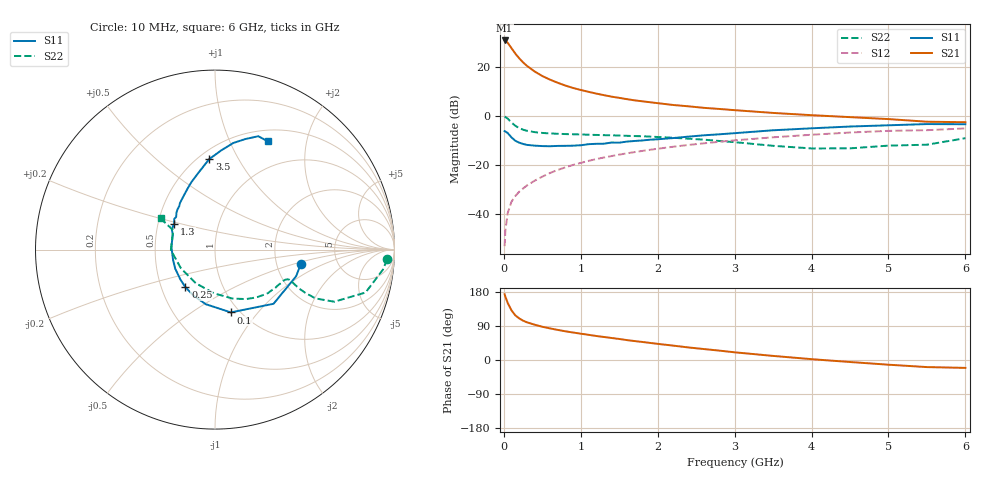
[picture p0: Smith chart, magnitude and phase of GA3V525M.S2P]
! Infineon Technologies  Discrete & RF Semiconductors
! BF775
! Si NPN RF Bipolar Junction Transistor in SOT23
! VCE = 3.5 V  IC = 25 mA
! Common Emitter S-Parameters:  May  1996
# GHz  S  MA  R  50
!  f  S11  S21  S12  S22
! GHz  MAG  ANG  MAG  ANG  MAG  ANG  MAG  ANG
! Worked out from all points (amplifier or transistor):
!   36 points, 10 MHz to 6 GHz, reference 50 ohm
!   highest |S21| = 30.7 dB at 10 MHz (marker M1)
!   |S21| within 3 dB of that: start of sweep to 96.53 MHz
!   unconditionally stable (mu >= 1): 321.8 MHz to 3.072 GHz
!   at 250 MHz: K = 0.93, MSG = 25.7 dB, |S12| = -29.7 dB
!   at 1.4 GHz: K = 1.12, MAG = 10.0 dB, |S12| = -16.4 dB
!   at 6 GHz: K = 0.96, MSG = 1.3 dB, |S12| = -5.2 dB
!   S11 on the Smith chart (normalised r, x): 10 MHz: 2.75, -0.57; 100 MHz: 0.91, -0.73; 250 MHz: 0.66, -0.30; 1.3 GHz: 0.61, +0.19; 3.5 GHz: 0.56, +0.76; 6 GHz: 0.64, +1.40
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0.01  0.4853 -9.4  34.16 173.5  0.0022 89.6  0.9608 -3.2
0.02  0.4757 -18.2  33.76 167.2  0.0046 85.9  0.9423 -6.8
0.05  0.4444 -42.8  30.65 150.6  0.0104 76.0  0.8724 -15.9
0.1  0.361 -75.8  23.76 130.8  0.0178 69.4  0.7253 -23.6
0.15  0.3086 -99.5  18.38 117.7  0.0232 66.4  0.6228 -25.9
0.2  0.2823 -115.6  14.78 109.7  0.0283 67.7  0.5598 -25.6
0.25  0.2661 -128.4  12.21 103.8  0.0329 68.3  0.5194 -24.9
0.3  0.2546 -139.3  10.39 99.5  0.0379 69.4  0.4938 -24.0
0.4  0.2458 -154.3  7.972 93.2  0.0474 70.9  0.4632 -22.7
0.5  0.2407 -166.0  6.436 87.7  0.0574 71.7  0.446 -22.1
0.6  0.2391 -174.3  5.436 83.4  0.0681 71.9  0.4357 -22.3
0.7  0.2426 177.3  4.695 79.4  0.0785 71.7  0.4286 -22.9
0.8  0.2434 171.7  4.116 75.8  0.0888 71.0  0.423 -23.7
0.9  0.2454 165.4  3.679 72.5  0.0994 70.6  0.4185 -24.4
1.1  0.2632 155.8  3.071 66.5  0.1202 69.1  0.4105 -27.3
1.3  0.269 147.6  2.627 60.8  0.1409 67.4  0.4019 -30.2
1.7  0.3059 133.2  2.056 50.0  0.1816 63.5  0.3852 -37.2
2.2  0.3505 119.2  1.656 38.0  0.2332 58.0  0.3556 -47.8
3.5  0.5054 93.6  1.14 10.8  0.3632 41.4  0.2438 -91.3
4.5  0.6025 80.3  0.936 -5.3  0.4546 27.5  0.2164 -151.3
5.5  0.6761 69.1  0.755 -18.7  0.5074 12.1  0.2568 155.2
6  0.6714 63.9  0.738 -20.8  0.5511 7.8  0.3488 150.2
